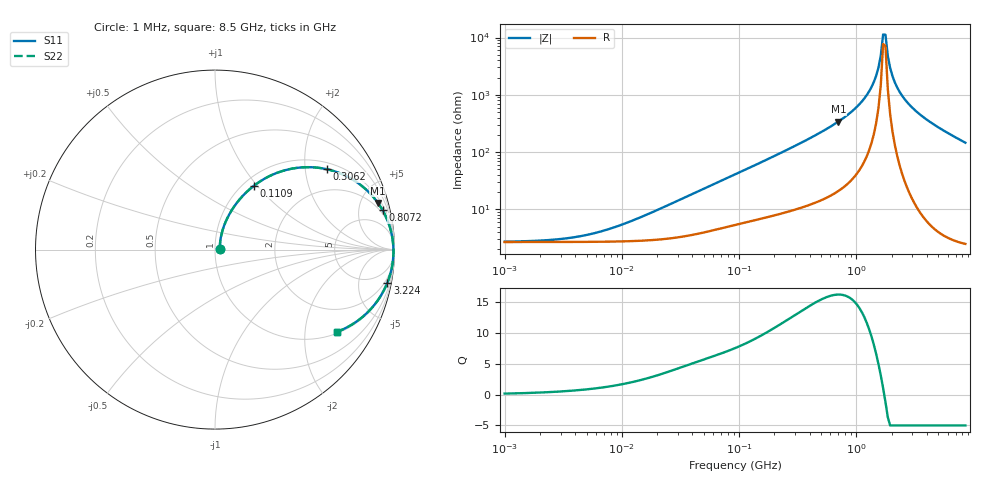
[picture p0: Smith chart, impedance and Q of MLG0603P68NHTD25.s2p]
! S-Parameter Data Generated by TDK Corporation
! Copyright(C) 2025 TDK Corporation.
! All Rights Reserved.
! TDK P/N: MLG0603P68NHTD25 (SMD / SMT Inductor (Coil))
! Property: L=68nH at 300MHz
! Size(LxWxT): 0.6x0.3x0.3mm
! Model Type: s2p (Touchstone File Format Version 1.0)
! Frequency: DC=Yes Start=1MHz Stop=8500MHz 198points Log-sweep
! Model Generated on Feb. 6, 2025
! Terms and conditions regarding TDK Simulation Models:
! 1)This simulation model is being provided solely for informational
!  purposes. Please refer to the specifications of the products in
!  terms of detailed characteristics of such products.
! 2)In no event shall TDK Corporation of any of its subsidiaries be
!  liable for any loss or damage arising, directly or indirectly,
!  from any information contained in this simulation model, including,
!  but not limited to loss or damages arising from any inaccuracies,
!  omissions or errors in connection with such information.
! 3)Any and all copyrights on this simulation model are owned by
!  TDK Corporation.  Duplication or redistribution of this simulation
!  model without prior written permission from TDK Corporation
!  is prohibited.
! 4)This simulation model is subject to any modification or change
!  without any prior notice.
! 5)Neither TDK Corporation nor any of its subsidiaries shall make any
!  warranty, express or implied, including but not limited to the
!  correctness, implied warranties of merchantability and fitness for
!  a particular purpose with respect to this simulation models.
! 6)The use of this simulation model shall be deemed to have consented
!  to the terms and conditions hereof.
! Port Assignments:
!  1 ---@@@--- 2
! Applicable Conditions:
!  Temperature = 25 degC
!  DC Bias Current = 0 A
!  Small Signal Operation
# Hz S MA R 50
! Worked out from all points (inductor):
!   197 points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, 1 MHz to 8.5 GHz, reference 50 ohm
!   read as one part in series: L = 73.6 nH near 19.19 MHz
!   highest Q = 16.3 at 702.8 MHz (marker M1), where L = 77.2 nH
!   self-resonance near 1.689 GHz
!   S11 on the Smith chart (normalised r, x): 1 MHz: 1.05, +0.01; 110.9 MHz: 1.12, +0.96; 306.2 MHz: 1.20, +2.62; 807.2 MHz: 1.52, +8.34; 3.224 GHz: 1, -10; 8.5 GHz: 1.05, -2.92
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1000000  0.02659 9.6  0.9738 -0.3  0.9738 -0.3  0.02659 9.6
4587603  0.03358 37.2  0.9735 -1.2  0.9735 -1.2  0.03358 37.2
2.10461e7  0.09857 67.6  0.9667 -5.4  0.9667 -5.4  0.09857 67.6
9.219544e7  0.361 61.5  0.8864 -21.0  0.8864 -21.0  0.361 61.5
1.108924e8  0.417 58.6  0.86 -24.5  0.86 -24.5  0.417 58.6
3.061674e8  0.7677 35.7  0.5849 -49.9  0.5849 -49.9  0.7677 35.7
4.229561e8  0.8557 27.5  0.4627 -58.6  0.4627 -58.6  0.8557 27.5
7.027873e8  0.9443 16.0  0.2763 -70.5  0.2763 -70.5  0.9443 16.0
8.071757e8  0.9591 13.2  0.2296 -73.2  0.2296 -73.2  0.9591 13.2
1.115076e9  0.9823 7.3  0.1279 -78.4  0.1279 -78.4  0.9823 7.3
1.404574e9  0.991 3.4  0.05998 -79.6  0.05998 -79.6  0.991 3.4
1.540426e9  0.9929 1.9  0.03359 -76.8  0.03359 -76.8  0.9929 1.9
1.613203e9  0.9935 1.1  0.02066 -71.2  0.02066 -71.2  0.9935 1.1
1.689417e9  0.994 0.4  0.008789 -46.8  0.008789 -46.8  0.994 0.4
1.769233e9  0.9943 -0.4  0.008881 49.6  0.008881 49.6  0.9943 -0.4
1.852819e9  0.9943 -1.2  0.02081 73.6  0.02081 73.6  0.9943 -1.2
1.940355e9  0.9942 -1.9  0.03382 79.1  0.03382 79.1  0.9942 -1.9
2.128028e9  0.9933 -3.5  0.06048 81.9  0.06048 81.9  0.9933 -3.5
2.333852e9  0.9916 -5.0  0.08771 82.0  0.08771 82.0  0.9916 -5.0
3.224109e9  0.9779 -10.9  0.1886 77.9  0.1886 77.9  0.9779 -10.9
4.884749e9  0.9367 -19.7  0.3365 69.5  0.3365 69.5  0.9367 -19.7
8.5e9  0.8183 -34.1  0.561 54.9  0.561 54.9  0.8183 -34.1
